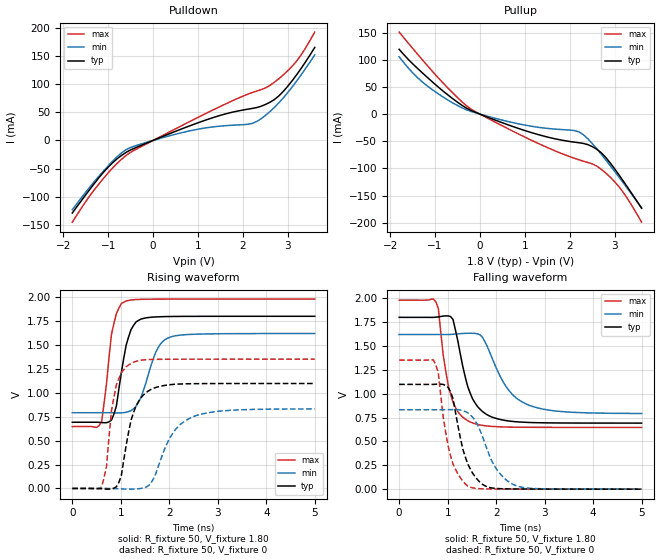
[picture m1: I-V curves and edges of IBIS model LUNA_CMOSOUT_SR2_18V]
[IBIS Ver]   3.2
[Comment Char]   |_char
[File name]   sg2520cbn_18v_c.ibs
[File Rev]   1.1
[Date]   2021/10/19 9:35:58
[Source]
[Notes]
[Disclaimer]
This information is for modeling purposes only, and is not guaranteed.
Property of SEIKO EPSON Corp.,
unauthorized reproduction and/or distribution is strictly prohibited.
[Copyright]
Copyright 2021, SEIKO EPSON Corp.
[Component]   2G005_2016
Si_location Pin
Timing_location Pin
[Manufacturer]   SEIKO EPSON Corp.
| 2016 PKG
[Package]
R_pkg   42m   NA   NA
L_pkg   0.49n   NA   NA
C_pkg   0.178p   NA   NA
[Pin] signal_name   model_name
1   OE   NC
2   GND   GND
3   OUT   LUNA_CMOSOUT_SR2_18V
4   VCC   POWER
| Models and submodels in the file (1): LUNA_CMOSOUT_SR2_18V (Output)
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[Model]   LUNA_CMOSOUT_SR2_18V
Model_type Output
Polarity Non-Inverting
Vmeas=0.90
C_comp   2.5p   2.0p   3.0p
[Temperature Range] 25   140   -40
[Voltage Range]   1.80   1.62   1.98
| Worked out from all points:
|   slope of the pulldown table from 0 to 0.27 V, typ, clamps not added: 30.6 ohm
|   slope of the pullup table from 0 to 0.27 V, typ, clamps not added: 30.8 ohm
|   falling waveform, R_fixture 50, V_fixture 1.80: 20-80 % time 354ps typ, 557ps min, 264ps max; typ from 1.8 V to 0.692 V
|   falling waveform, R_fixture 50, V_fixture 0: 20-80 % time 323ps typ, 447ps min, 269ps max; typ from 1.1 V to 0 V
|   rising waveform, R_fixture 50, V_fixture 1.80: 20-80 % time 233ps typ, 332ps min, 193ps max; typ from 0.692 V to 1.8 V
|   rising waveform, R_fixture 50, V_fixture 0: 20-80 % time 294ps typ, 491ps min, 196ps max; typ from 0 V to 1.1 V
[Pullup]
-1.8V     119.3mA    105.5mA    151mA
-1.5V     92.77mA    76.17mA    121.1mA
-1.2V     69.69mA    53.54mA    92.04mA
-600mV    28.04mA    20.35mA    38.49mA
-200mV    6.819mA    4.987mA    9.213mA
1.2V      -35.35mA   -23mA      -50.19mA
2.1V      -51.55mA   -30.23mA   -81.18mA
2.3V      -53.88mA   -37.68mA   -86.56mA
2.7V      -71mA      -73.76mA   -101.5mA
3V        -100.8mA   -105.6mA   -124.5mA
3.3V      -136.3mA   -138.6mA   -157.4mA
3.6V      -173.3mA   -172.5mA   -198.9mA
[Pulldown]
-1.8V     -129.2mA   -123.3mA   -145.5mA
-1.4V     -86.11mA   -82.03mA   -97.49mA
-1.1V     -56.21mA   -54.04mA   -67.06mA
-600mV    -21.19mA   -16.39mA   -26.56mA
300mV     9.791mA    6.802mA    12.4mA
1.2V      36.97mA    22.63mA    48.89mA
2.1V      55.44mA    28.57mA    81.94mA
2.4V      60.61mA    38.22mA    90.17mA
2.8V      79.1mA     66.85mA    109.8mA
3.1V      106.5mA    95.36mA    132.2mA
3.3V      128.5mA    117mA      152.6mA
3.6V      165.4mA    152.2mA    192.7mA
[Falling Waveform]
R_fixture=50
V_fixture=1.80
V_fixture_min=1.62
V_fixture_max=1.98
0s        1.8V       1.62V      1.98V
757.6ps   1.802V     1.62V      1.96V
808.1ps   1.805V     1.62V      1.894V
909.1ps   1.813V     1.619V     1.403V
1.061ns   1.808V     1.621V     995.7mV
1.414ns   1.075V     1.633V     717.6mV
1.818ns   778.3mV    1.493V     661.8mV
2.222ns   717mV      1.062V     650.7mV
2.626ns   700mV      890.8mV    648.3mV
5ns       692.2mV    793mV      647.3mV
[Falling Waveform]
R_fixture=50
V_fixture=0
V_fixture_min=0
V_fixture_max=0
0s        1.098V     831.9mV    1.352V
707.1ps   1.097V     831.8mV    1.353V
808.1ps   1.101V     831.7mV    1.216V
909.1ps   1.097V     831.7mV    754.8mV
1.061ns   1.018V     833.3mV    350.4mV
1.414ns   266mV      800.3mV    32.8mV
1.768ns   35.83mV    481.8mV    3.384mV
2.02ns    7.051mV    200.1mV    1.78mV
2.374ns   2.546mV    44.88mV    1.095mV
5ns       425.5uV    849.4uV    233.6uV
[Rising Waveform]
R_fixture=50
V_fixture=1.80
V_fixture_min=1.62
V_fixture_max=1.98
0s        692.1mV    791.8mV    647.3mV
606.1ps   689mV      792.1mV    700.4mV
808.1ps   714.9mV    791.2mV    1.61V
909.1ps   860.8mV    789.6mV    1.828V
1.061ns   1.36V      792.9mV    1.947V
1.212ns   1.661V     814.1mV    1.971V
1.313ns   1.74V      857.5mV    1.975V
1.717ns   1.793V     1.419V     1.979V
2.02ns    1.798V     1.583V     1.98V
5ns       1.8V       1.62V      1.98V
[Rising Waveform]
R_fixture=50
V_fixture=0
V_fixture_min=0
V_fixture_max=0
0s        14.57nV    396.7nV    14.6nV
606.1ps   -2.597mV   186.8uV    17.21mV
707.1ps   -6.824mV   471.2uV    238.1mV
808.1ps   -5.392mV   -157.5uV   810.3mV
909.1ps   17.71mV    -2.055mV   1.083V
1.212ns   714.4mV    -7.231mV   1.308V
1.616ns   1.034V     50.83mV    1.348V
2.02ns    1.085V     535.8mV    1.351V
2.475ns   1.095V     746.6mV    1.352V
5ns       1.098V     831.4mV    1.352V
[Ramp]
R_load=50
dV/dt_r   6.586E-1/2.940E-10   4.988E-1/4.900E-10   8.111E-1/1.958E-10
dV/dt_f   6.647E-1/3.522E-10   4.962E-1/5.533E-10   7.996E-1/2.618E-10
|[End   LUNA_CMOSOUT_SR2_18V
